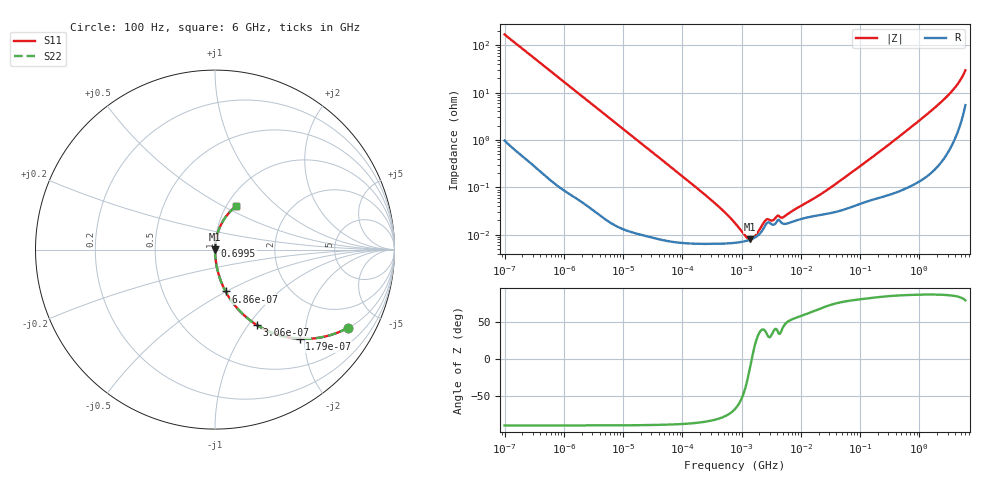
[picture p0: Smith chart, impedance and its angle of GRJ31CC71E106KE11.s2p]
!Murata Part Number: GRJ31CC71E106KE11
!These Parameters are Measured in Series Mode Connection
!Data Generated on Jun 19, 2026
!  o--ll--o
!Port1  Port2
!  o------o
!Operation Temp=25[degC], DC Bias Voltage=0[V]
!Freq. Start=100[Hz] Stop=6[GHz] 401[Steps]
# Hz S RI R 50
!Freq.(Hz) S11(Real) S11(Imag) S21(Real) S21(Imag) S12(Real) S12(Imag) S22(Real) S22(Imag)
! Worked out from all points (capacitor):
!   401 points, 100 Hz to 6 GHz, reference 50 ohm
!   read as one part in series: C = 9.41 uF near 109 Hz
!   lowest |Z| = 8.01 mohm at 1.386 MHz (marker M1)
!   series resonance near 1.485 MHz, so ESL is about 1.2 nH
!   S11 on the Smith chart (normalised r, x): 100 Hz: 1.02, -3.38; 179 Hz: 1.01, -1.89; 306 Hz: 1.01, -1.11; 686 Hz: 1.00, -0.50; 699.5 MHz: 1.00, +0.04; 6 GHz: 1.11, +0.58
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100  0.7392 -0.4362  0.2608 0.4362  0.2608 0.4362  0.7392 -0.4362
179  0.472 -0.4965  0.528 0.4965  0.528 0.4965  0.472 -0.4965
306  0.2356 -0.4217  0.7644 0.4217  0.7644 0.4217  0.2356 -0.4217
686  0.0588 -0.2329  0.9412 0.2329  0.9412 0.2329  0.0588 -0.2329
2008  0.00763 -0.0842  0.9924 0.0842  0.9924 0.0842  0.00763 -0.0842
40335  9.83e-05 -0.00426  0.9999 0.00426  0.9999 0.00426  9.83e-05 -0.00426
316350  6.43e-05 -0.000521  0.9999 0.000521  0.9999 0.000521  6.43e-05 -0.000521
774597  6.75e-05 -0.000163  0.9999 0.000163  0.9999 0.000163  6.75e-05 -0.000163
1108252  7.24e-05 -6.98e-05  0.9999 6.98e-05  0.9999 6.98e-05  7.24e-05 -6.98e-05
1386327  7.84e-05 -1.63e-05  0.9999 1.63e-05  0.9999 1.63e-05  7.84e-05 -1.63e-05
1813585  9.3e-05 4.9e-05  0.9999 -4.9e-05  0.9999 -4.9e-05  9.3e-05 4.9e-05
2594782  0.000168 0.000121  0.9998 -0.000121  0.9998 -0.000121  0.000168 0.000121
3245845  0.000165 0.000109  0.9998 -0.000109  0.9998 -0.000109  0.000165 0.000109
4060267  0.000201 0.000156  0.9998 -0.000156  0.9998 -0.000156  0.000201 0.000156
5079039  0.00017 0.000163  0.9998 -0.000163  0.9998 -0.000163  0.00017 0.000163
1.555665e7  0.000243 0.000498  0.9998 -0.000498  0.9998 -0.000498  0.000243 0.000498
3.983537e7  0.000306 0.00117  0.9997 -0.00117  0.9997 -0.00117  0.000306 0.00117
3.124326e8  0.000761 0.00812  0.9992 -0.00812  0.9992 -0.00812  0.000761 0.00812
6.994765e8  0.00136 0.0179  0.9986 -0.0179  0.9986 -0.0179  0.00136 0.0179
2.931063e9  0.0117 0.0815  0.9883 -0.0815  0.9883 -0.0815  0.0117 0.0815
4.586474e9  0.0397 0.1509  0.9603 -0.1509  0.9603 -0.1509  0.0397 0.1509
6e9  0.1187 0.2431  0.8813 -0.2431  0.8813 -0.2431  0.1187 0.2431
